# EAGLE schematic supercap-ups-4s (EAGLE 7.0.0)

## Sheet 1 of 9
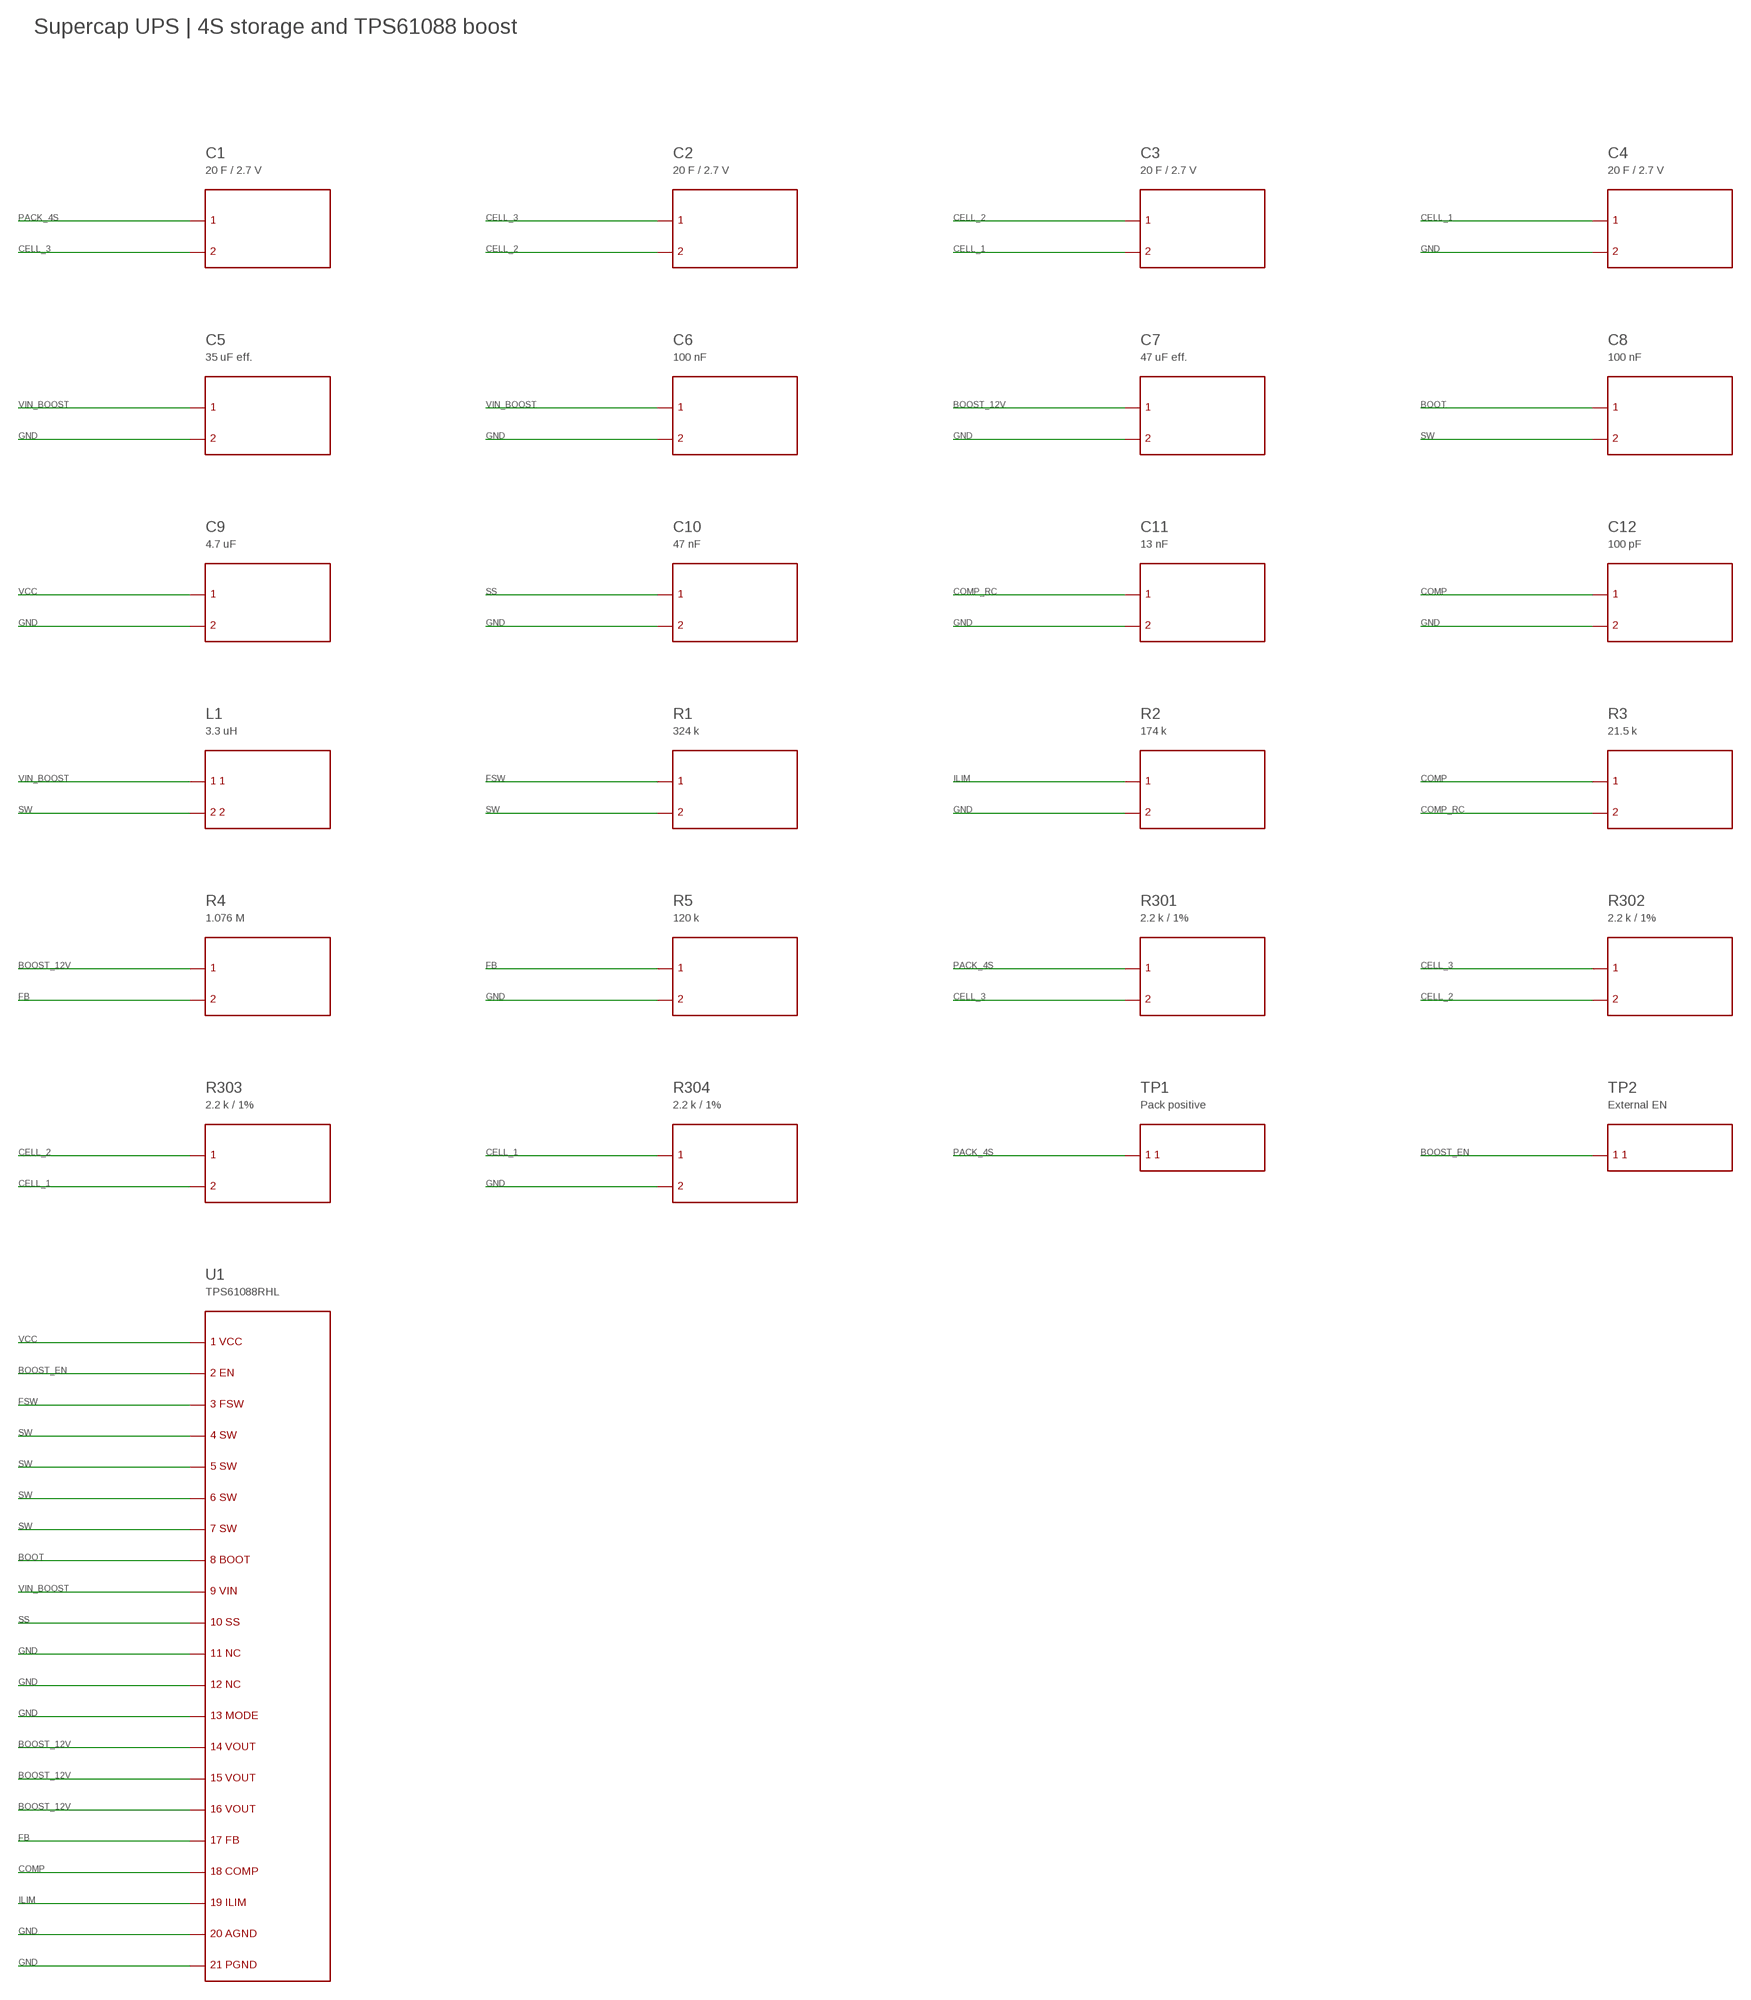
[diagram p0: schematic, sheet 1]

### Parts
C1  20 F / 2.7 V  SYM12  (no package)
C2  20 F / 2.7 V  SYM12  (no package)
C3  20 F / 2.7 V  SYM12  (no package)
C4  20 F / 2.7 V  SYM12  (no package)
C5  35 uF eff.  SYM11  (no package)
C6  100 nF  SYM11  (no package)
C7  47 uF eff.  SYM11  (no package)
C8  100 nF  SYM11  (no package)
C9  4.7 uF  SYM11  (no package)
C10  47 nF  SYM11  (no package)
C11  13 nF  SYM11  (no package)
C12  100 pF  SYM11  (no package)
L1  3.3 uH  SYM14  (no package)
R1  324 k  SYM15  (no package)
R2  174 k  SYM15  (no package)
R3  21.5 k  SYM15  (no package)
R4  1.076 M  SYM15  (no package)
R5  120 k  SYM15  (no package)
R301  2.2 k / 1%  SYM15  (no package)
R302  2.2 k / 1%  SYM15  (no package)
R303  2.2 k / 1%  SYM15  (no package)
R304  2.2 k / 1%  SYM15  (no package)
TP1  Pack positive  SYM8  (no package)
TP2  External EN  SYM8  (no package)
U1  TPS61088RHL  SYM25  (no package)

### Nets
BOOST_12V: C7.P1 R4.P1 U1.P14 U1.P15 U1.P16
BOOST_EN: TP2.P1 U1.P2 ; also sheet 9
BOOT: C8.P1 U1.P8
CELL_1: C3.P2 C4.P1 R303.P2 R304.P1 ; also sheet 4,8
CELL_2: C2.P2 C3.P1 R302.P2 R303.P1 ; also sheet 4,8
CELL_3: C1.P2 C2.P1 R301.P2 R302.P1 ; also sheet 4,8
COMP: C12.P1 R3.P1 U1.P18
COMP_RC: C11.P1 R3.P2
FB: R4.P2 R5.P1 U1.P17
FSW: R1.P1 U1.P3
GND: C4.P2 C5.P2 C6.P2 C7.P2 C9.P2 C10.P2 C11.P2 C12.P2 R2.P2 R5.P2 R304.P2 U1.P11 U1.P12 U1.P13 U1.P20 U1.P21 ; also sheet 2,3,4,5,6,7,8,9
ILIM: R2.P1 U1.P19
PACK_4S: C1.P1 R301.P1 TP1.P1 ; also sheet 2,3,4,5,6,8
SS: C10.P1 U1.P10
SW: C8.P2 L1.P2 R1.P2 U1.P4 U1.P5 U1.P6 U1.P7
VCC: C9.P1 U1.P1
VIN_BOOST: C5.P1 C6.P1 L1.P1 U1.P9 ; also sheet 5

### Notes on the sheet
- Supercap UPS | 4S storage and TPS61088 boost

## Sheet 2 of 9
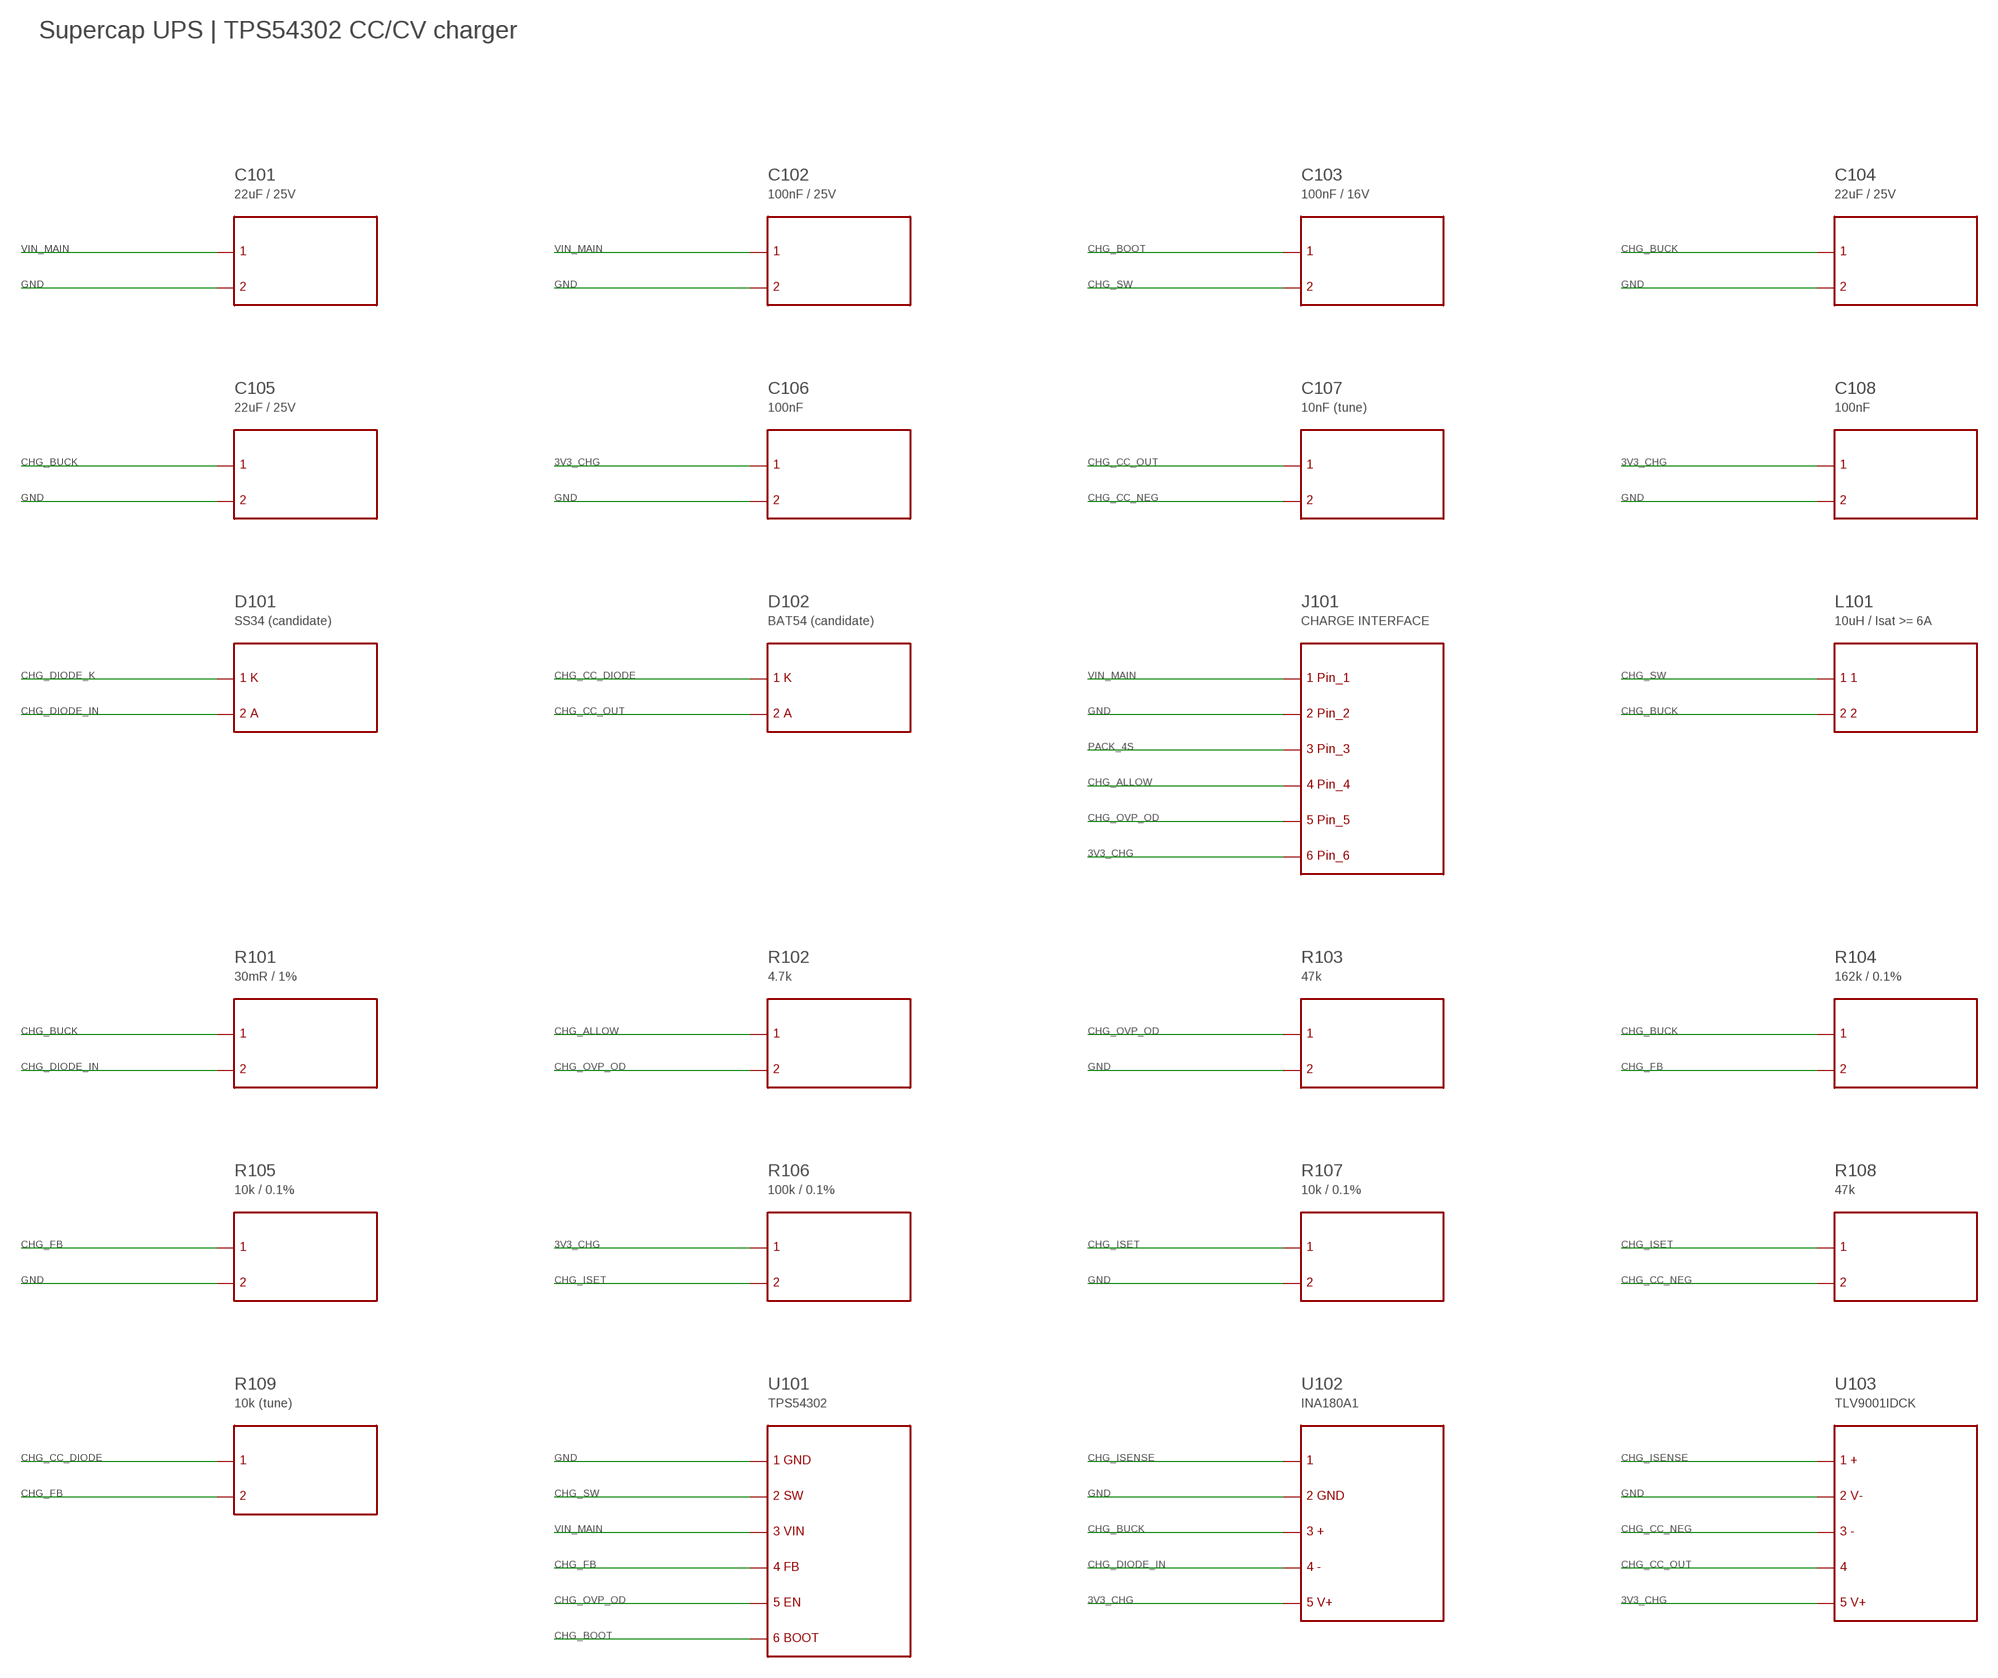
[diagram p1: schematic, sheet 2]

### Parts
C101  22uF / 25V  SYM11  (no package)
C102  100nF / 25V  SYM11  (no package)
C103  100nF / 16V  SYM11  (no package)
C104  22uF / 25V  SYM11  (no package)
C105  22uF / 25V  SYM11  (no package)
C106  100nF  SYM11  (no package)
C107  10nF (tune)  SYM11  (no package)
C108  100nF  SYM11  (no package)
D101  SS34 (candidate)  SYM13  (no package)
D102  BAT54 (candidate)  SYM13  (no package)
J101  CHARGE INTERFACE  SYM9  (no package)
L101  10uH / Isat >= 6A  SYM14  (no package)
R101  30mR / 1%  SYM15  (no package)
R102  4.7k  SYM15  (no package)
R103  47k  SYM15  (no package)
R104  162k / 0.1%  SYM15  (no package)
R105  10k / 0.1%  SYM15  (no package)
R106  100k / 0.1%  SYM15  (no package)
R107  10k / 0.1%  SYM15  (no package)
R108  47k  SYM15  (no package)
R109  10k (tune)  SYM15  (no package)
U101  TPS54302  SYM24  (no package)
U102  INA180A1  SYM0  (no package)
U103  TLV9001IDCK  SYM3  (no package)

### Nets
3V3_CHG: C106.P1 C108.P1 J101.P6 R106.P1 U102.P5 U103.P5 ; also sheet 7
CHG_ALLOW: J101.P4 R102.P1
CHG_BOOT: C103.P1 U101.P6
CHG_BUCK: C104.P1 C105.P1 L101.P2 R101.P1 R104.P1 U102.P3
CHG_CC_DIODE: D102.P1 R109.P1
CHG_CC_NEG: C107.P2 R108.P2 U103.P3
CHG_CC_OUT: C107.P1 D102.P2 U103.P4
CHG_DIODE_IN: D101.P2 R101.P2 U102.P4
CHG_DIODE_K: D101.P1 ; also sheet 6
CHG_FB: R104.P2 R105.P1 R109.P2 U101.P4 ; also sheet 6
CHG_ISENSE: U102.P1 U103.P1
CHG_ISET: R106.P2 R107.P1 R108.P1
CHG_OVP_OD: J101.P5 R102.P2 R103.P1 U101.P5 ; also sheet 4,7
CHG_SW: C103.P2 L101.P1 U101.P2
GND: C101.P2 C102.P2 C104.P2 C105.P2 C106.P2 C108.P2 J101.P2 R103.P2 R105.P2 R107.P2 U101.P1 U102.P2 U103.P2 ; also sheet 1,3,4,5,6,7,8,9
PACK_4S: J101.P3 ; also sheet 1,3,4,5,6,8
VIN_MAIN: C101.P1 C102.P1 J101.P1 U101.P3 ; also sheet 4,7

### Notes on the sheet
- Supercap UPS | TPS54302 CC/CV charger

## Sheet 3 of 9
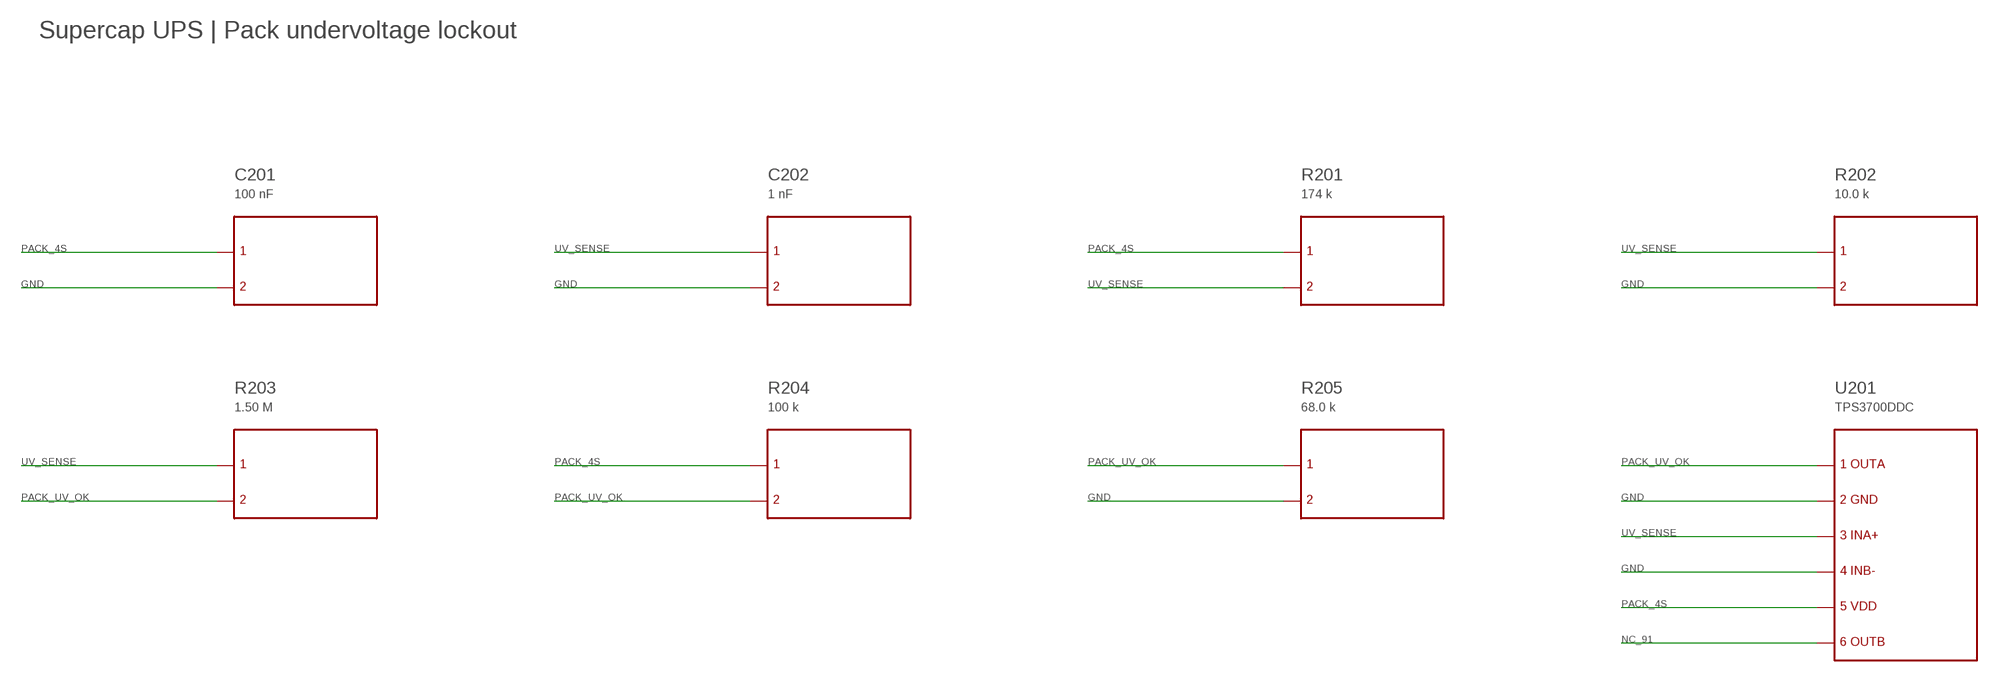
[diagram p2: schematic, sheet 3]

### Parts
C201  100 nF  SYM11  (no package)
C202  1 nF  SYM11  (no package)
R201  174 k  SYM15  (no package)
R202  10.0 k  SYM15  (no package)
R203  1.50 M  SYM15  (no package)
R204  100 k  SYM15  (no package)
R205  68.0 k  SYM15  (no package)
U201  TPS3700DDC  SYM29  (no package)

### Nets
GND: C201.P2 C202.P2 R202.P2 R205.P2 U201.P2 U201.P4 ; also sheet 1,2,4,5,6,7,8,9
NC_91: U201.P6
PACK_4S: C201.P1 R201.P1 R204.P1 U201.P5 ; also sheet 1,2,4,5,6,8
PACK_UV_OK: R203.P2 R204.P2 R205.P1 U201.P1 ; also sheet 5,9
UV_SENSE: C202.P1 R201.P2 R202.P1 R203.P1 U201.P3

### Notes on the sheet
- Supercap UPS | Pack undervoltage lockout

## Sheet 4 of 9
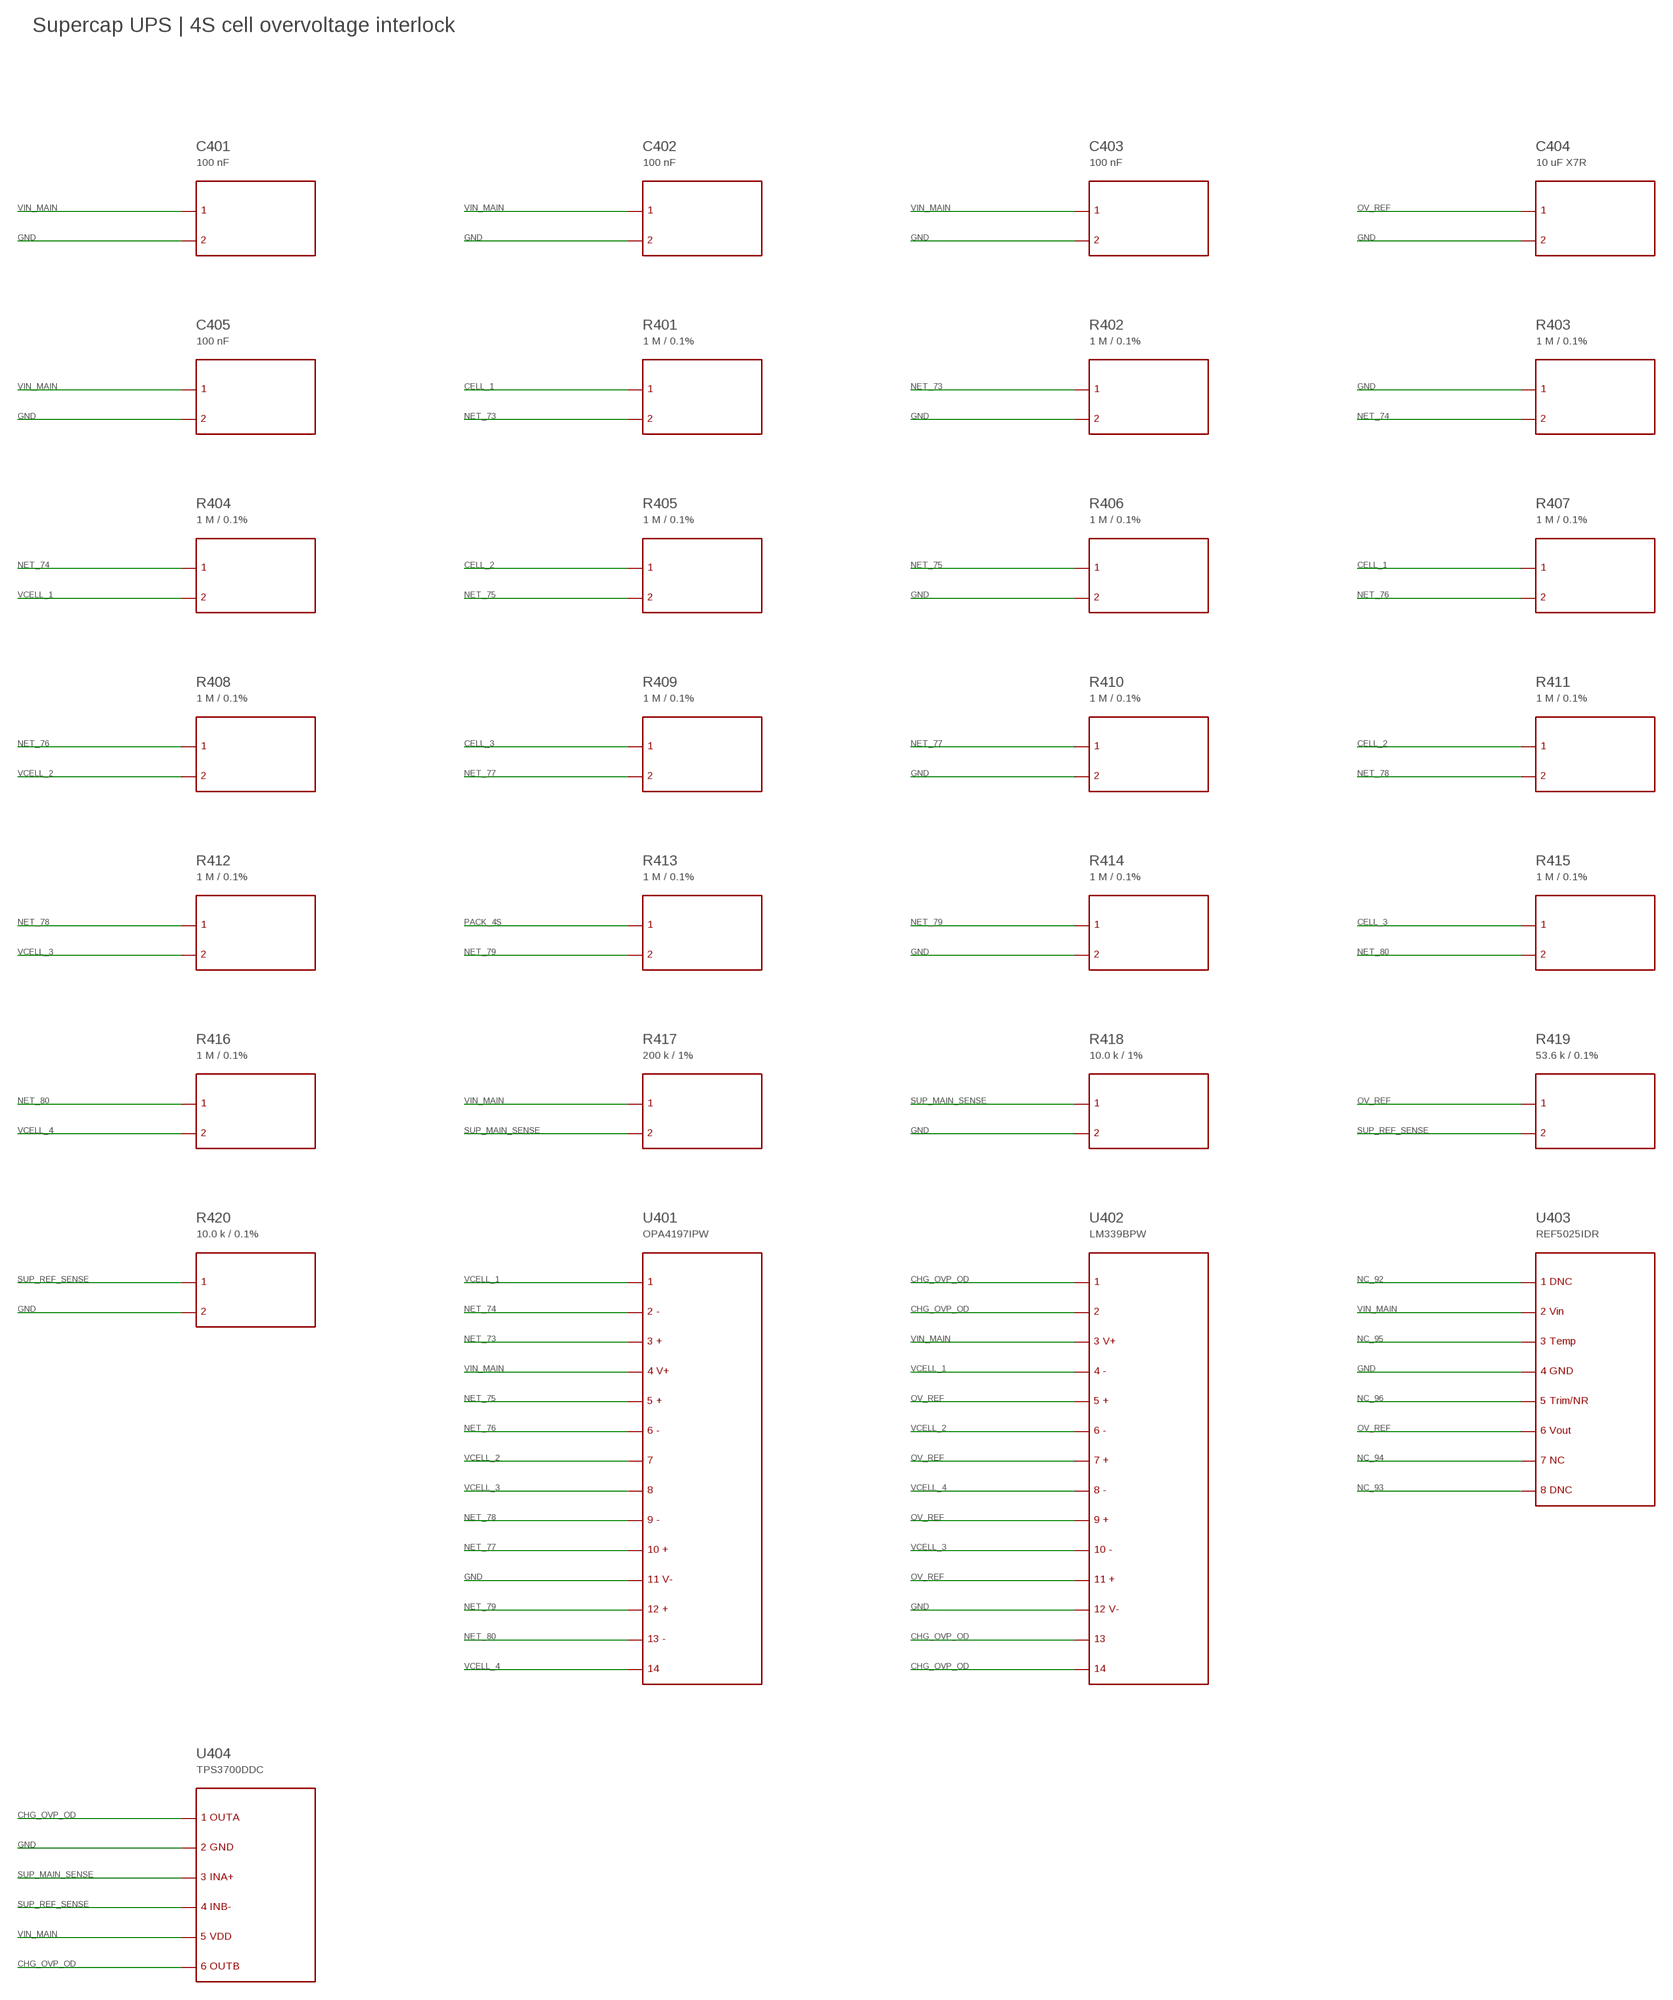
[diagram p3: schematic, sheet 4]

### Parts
C401  100 nF  SYM11  (no package)
C402  100 nF  SYM11  (no package)
C403  100 nF  SYM11  (no package)
C404  10 uF X7R  SYM11  (no package)
C405  100 nF  SYM11  (no package)
R401  1 M / 0.1%  SYM15  (no package)
R402  1 M / 0.1%  SYM15  (no package)
R403  1 M / 0.1%  SYM15  (no package)
R404  1 M / 0.1%  SYM15  (no package)
R405  1 M / 0.1%  SYM15  (no package)
R406  1 M / 0.1%  SYM15  (no package)
R407  1 M / 0.1%  SYM15  (no package)
R408  1 M / 0.1%  SYM15  (no package)
R409  1 M / 0.1%  SYM15  (no package)
R410  1 M / 0.1%  SYM15  (no package)
R411  1 M / 0.1%  SYM15  (no package)
R412  1 M / 0.1%  SYM15  (no package)
R413  1 M / 0.1%  SYM15  (no package)
R414  1 M / 0.1%  SYM15  (no package)
R415  1 M / 0.1%  SYM15  (no package)
R416  1 M / 0.1%  SYM15  (no package)
R417  200 k / 1%  SYM15  (no package)
R418  10.0 k / 1%  SYM15  (no package)
R419  53.6 k / 0.1%  SYM15  (no package)
R420  10.0 k / 0.1%  SYM15  (no package)
U401  OPA4197IPW  SYM2  (no package)
U402  LM339BPW  SYM5  (no package)
U403  REF5025IDR  SYM6  (no package)
U404  TPS3700DDC  SYM7  (no package)

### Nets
CELL_1: R401.P1 R407.P1 ; also sheet 1,8
CELL_2: R405.P1 R411.P1 ; also sheet 1,8
CELL_3: R409.P1 R415.P1 ; also sheet 1,8
CHG_OVP_OD: U402.P1 U402.P2 U402.P13 U402.P14 U404.P1 U404.P6 ; also sheet 2,7
GND: C401.P2 C402.P2 C403.P2 C404.P2 C405.P2 R402.P2 R403.P1 R406.P2 R410.P2 R414.P2 R418.P2 R420.P2 U401.P11 U402.P12 U403.P4 U404.P2 ; also sheet 1,2,3,5,6,7,8,9
NC_92: U403.P1
NC_93: U403.P8
NC_94: U403.P7
NC_95: U403.P3
NC_96: U403.P5
NET_73: R401.P2 R402.P1 U401.P3
NET_74: R403.P2 R404.P1 U401.P2
NET_75: R405.P2 R406.P1 U401.P5
NET_76: R407.P2 R408.P1 U401.P6
NET_77: R409.P2 R410.P1 U401.P10
NET_78: R411.P2 R412.P1 U401.P9
NET_79: R413.P2 R414.P1 U401.P12
NET_80: R415.P2 R416.P1 U401.P13
OV_REF: C404.P1 R419.P1 U402.P5 U402.P7 U402.P9 U402.P11 U403.P6
PACK_4S: R413.P1 ; also sheet 1,2,3,5,6,8
SUP_MAIN_SENSE: R417.P2 R418.P1 U404.P3
SUP_REF_SENSE: R419.P2 R420.P1 U404.P4
VCELL_1: R404.P2 U401.P1 U402.P4
VCELL_2: R408.P2 U401.P7 U402.P6
VCELL_3: R412.P2 U401.P8 U402.P10
VCELL_4: R416.P2 U401.P14 U402.P8
VIN_MAIN: C401.P1 C402.P1 C403.P1 C405.P1 R417.P1 U401.P4 U402.P3 U403.P2 U404.P5 ; also sheet 2,7

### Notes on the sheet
- Supercap UPS | 4S cell overvoltage interlock

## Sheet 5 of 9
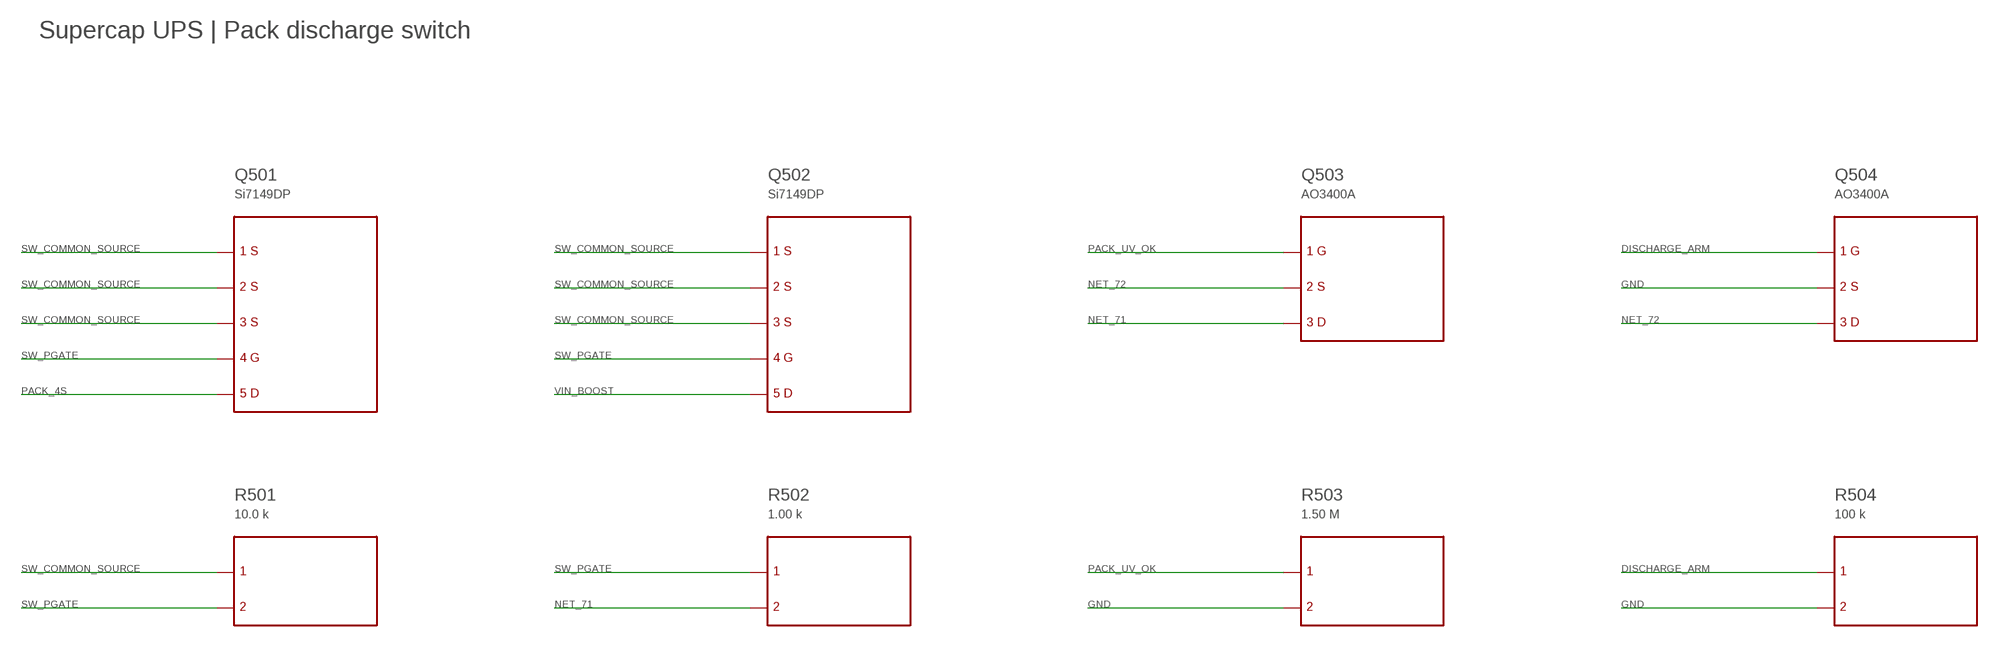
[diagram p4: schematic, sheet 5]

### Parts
Q501  Si7149DP  SYM32  (no package)
Q502  Si7149DP  SYM32  (no package)
Q503  AO3400A  SYM28  (no package)
Q504  AO3400A  SYM28  (no package)
R501  10.0 k  SYM15  (no package)
R502  1.00 k  SYM15  (no package)
R503  1.50 M  SYM15  (no package)
R504  100 k  SYM15  (no package)

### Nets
DISCHARGE_ARM: Q504.P1 R504.P1 ; also sheet 9
GND: Q504.P2 R503.P2 R504.P2 ; also sheet 1,2,3,4,6,7,8,9
NET_71: Q503.P3 R502.P2
NET_72: Q503.P2 Q504.P3
PACK_4S: Q501.P5 ; also sheet 1,2,3,4,6,8
PACK_UV_OK: Q503.P1 R503.P1 ; also sheet 3,9
SW_COMMON_SOURCE: Q501.P1 Q501.P2 Q501.P3 Q502.P1 Q502.P2 Q502.P3 R501.P1
SW_PGATE: Q501.P4 Q502.P4 R501.P2 R502.P1
VIN_BOOST: Q502.P5 ; also sheet 1

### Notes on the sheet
- Supercap UPS | Pack discharge switch

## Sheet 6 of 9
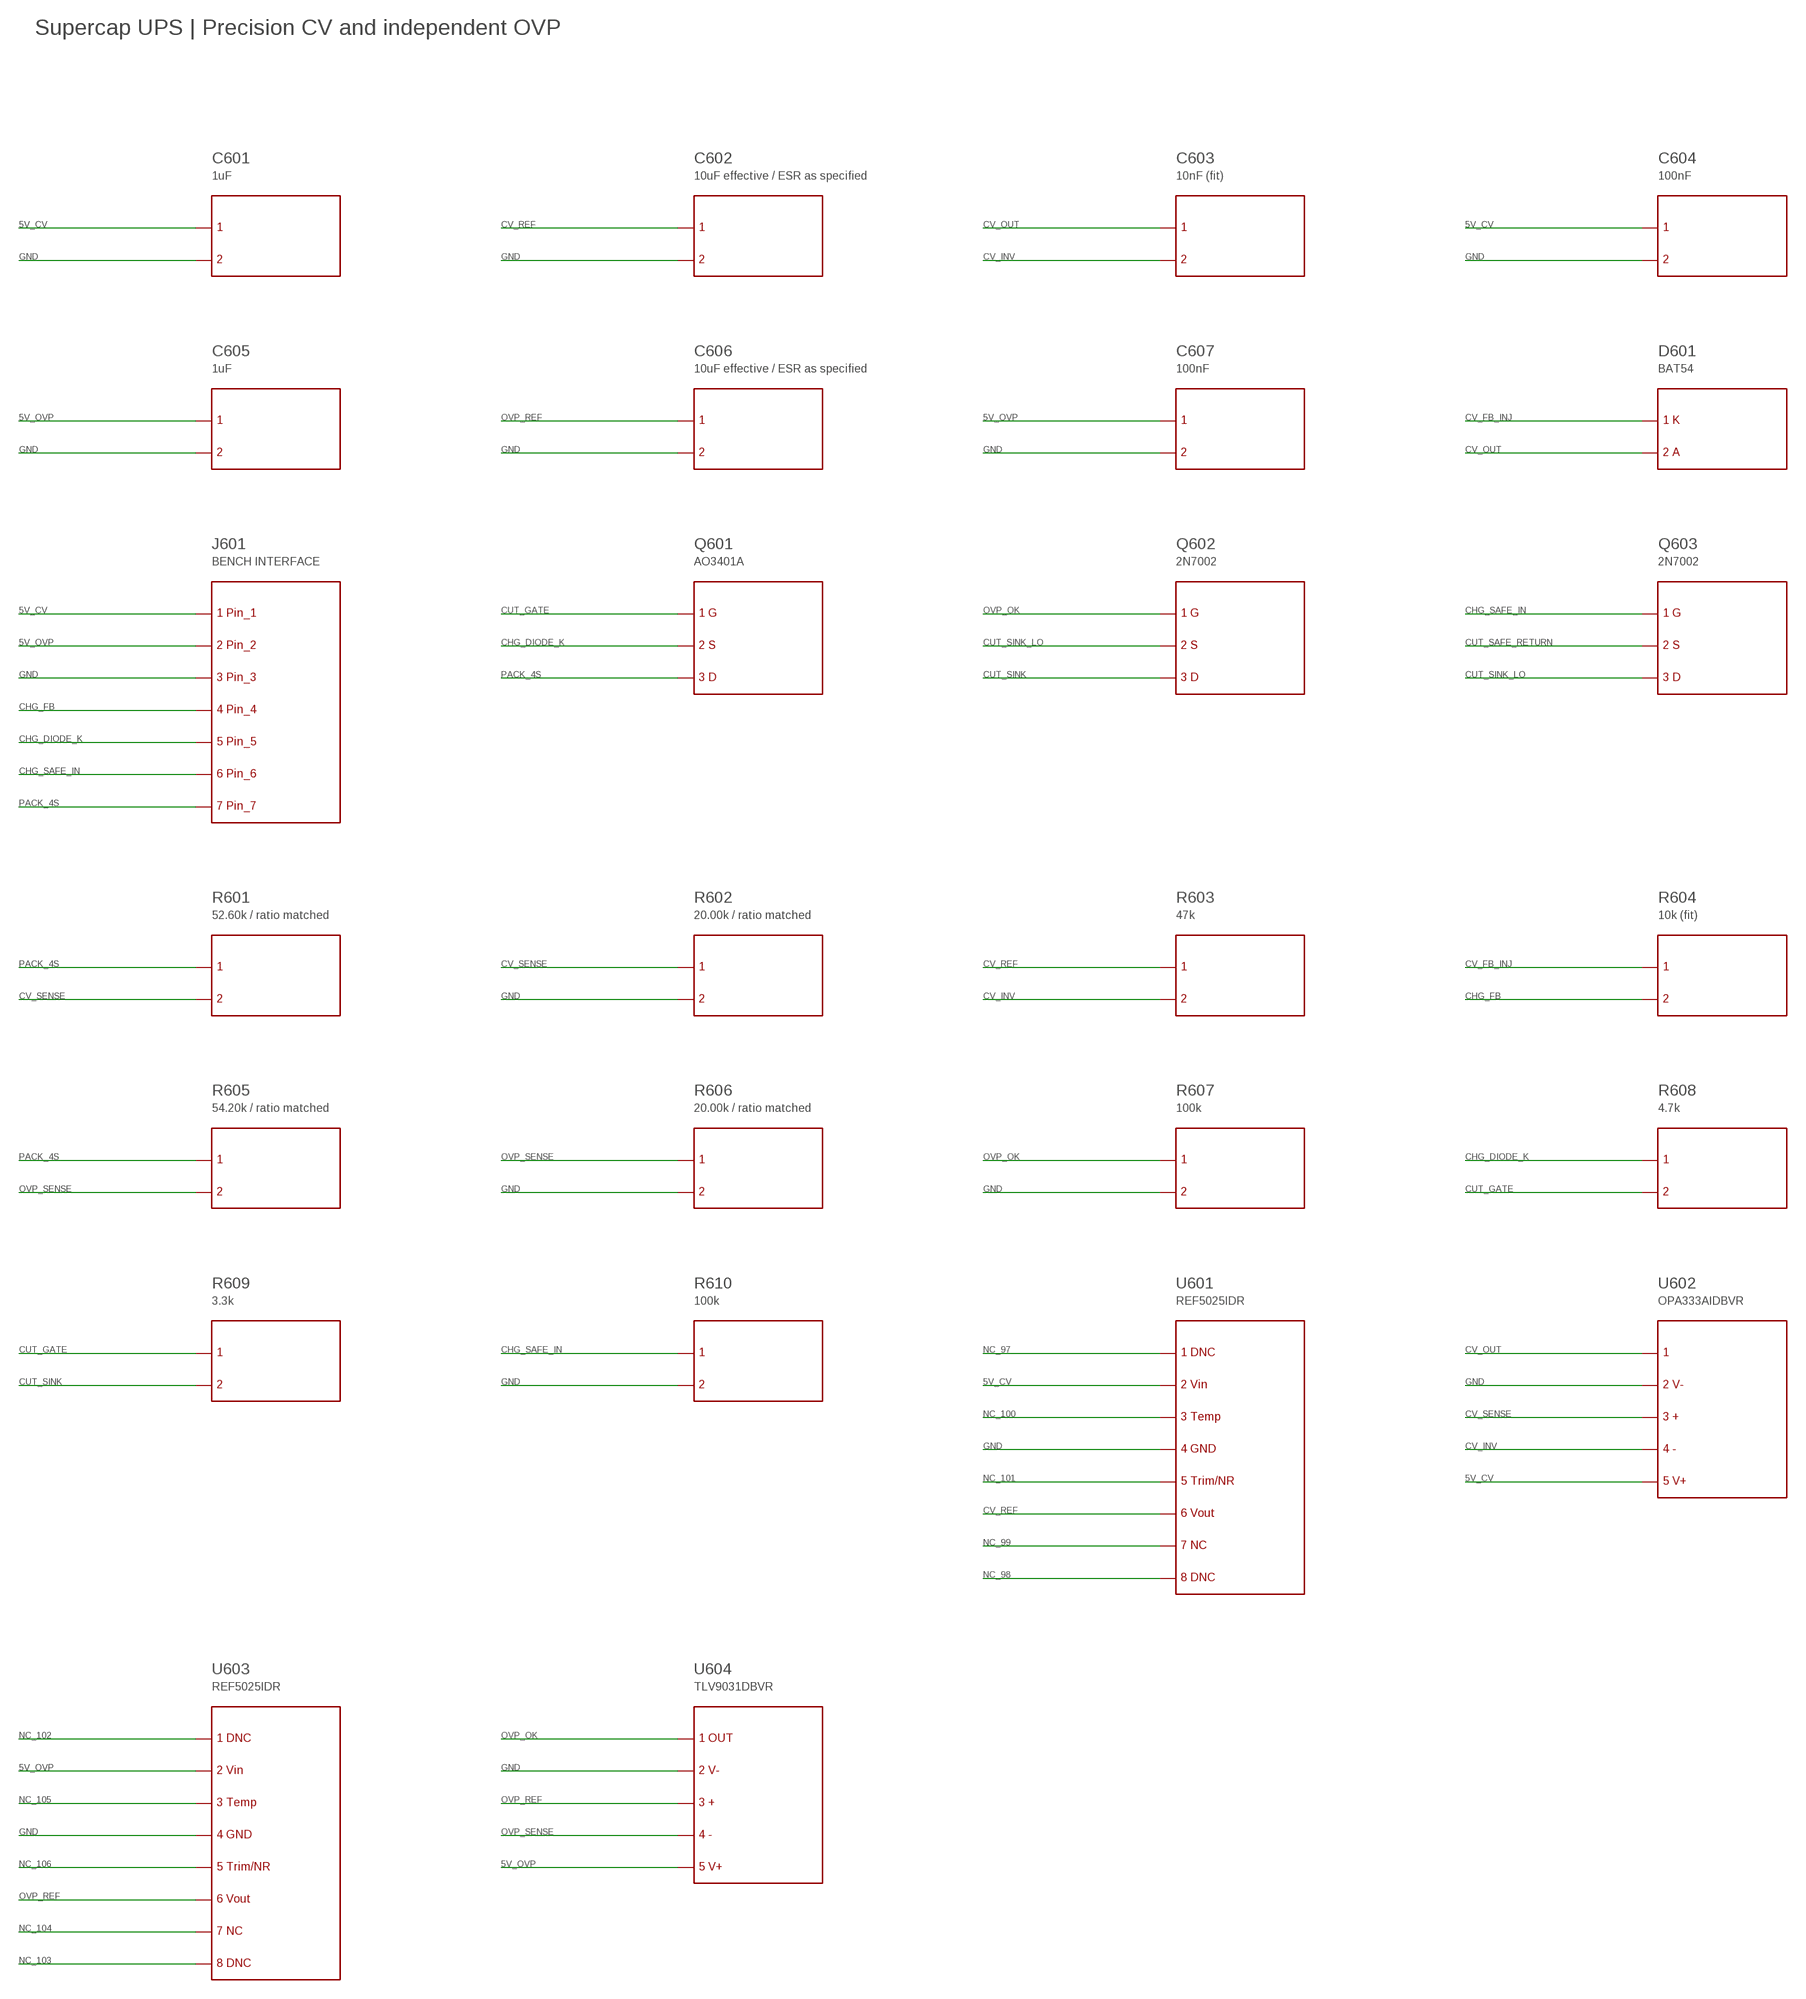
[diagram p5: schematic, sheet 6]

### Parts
C601  1uF  SYM11  (no package)
C602  10uF effective / ESR as specified  SYM11  (no package)
C603  10nF (fit)  SYM11  (no package)
C604  100nF  SYM11  (no package)
C605  1uF  SYM11  (no package)
C606  10uF effective / ESR as specified  SYM11  (no package)
C607  100nF  SYM11  (no package)
D601  BAT54  SYM13  (no package)
J601  BENCH INTERFACE  SYM10  (no package)
Q601  AO3401A  SYM27  (no package)
Q602  2N7002  SYM26  (no package)
Q603  2N7002  SYM26  (no package)
R601  52.60k / ratio matched  SYM15  (no package)
R602  20.00k / ratio matched  SYM15  (no package)
R603  47k  SYM15  (no package)
R604  10k (fit)  SYM15  (no package)
R605  54.20k / ratio matched  SYM15  (no package)
R606  20.00k / ratio matched  SYM15  (no package)
R607  100k  SYM15  (no package)
R608  4.7k  SYM15  (no package)
R609  3.3k  SYM15  (no package)
R610  100k  SYM15  (no package)
U601  REF5025IDR  SYM23  (no package)
U602  OPA333AIDBVR  SYM1  (no package)
U603  REF5025IDR  SYM23  (no package)
U604  TLV9031DBVR  SYM22  (no package)

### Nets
5V_CV: C601.P1 C604.P1 J601.P1 U601.P2 U602.P5 ; also sheet 7
5V_OVP: C605.P1 C607.P1 J601.P2 U603.P2 U604.P5 ; also sheet 7
CHG_DIODE_K: J601.P5 Q601.P2 R608.P1 ; also sheet 2
CHG_FB: J601.P4 R604.P2 ; also sheet 2
CHG_SAFE_IN: J601.P6 Q603.P1 R610.P1
CUT_GATE: Q601.P1 R608.P2 R609.P1
CUT_SAFE_RETURN: Q603.P2 ; also sheet 7
CUT_SINK: Q602.P3 R609.P2
CUT_SINK_LO: Q602.P2 Q603.P3
CV_FB_INJ: D601.P1 R604.P1
CV_INV: C603.P2 R603.P2 U602.P4
CV_OUT: C603.P1 D601.P2 U602.P1
CV_REF: C602.P1 R603.P1 U601.P6
CV_SENSE: R601.P2 R602.P1 U602.P3
GND: C601.P2 C602.P2 C604.P2 C605.P2 C606.P2 C607.P2 J601.P3 R602.P2 R606.P2 R607.P2 R610.P2 U601.P4 U602.P2 U603.P4 U604.P2 ; also sheet 1,2,3,4,5,7,8,9
NC_97: U601.P1
NC_98: U601.P8
NC_99: U601.P7
NC_100: U601.P3
NC_101: U601.P5
NC_102: U603.P1
NC_103: U603.P8
NC_104: U603.P7
NC_105: U603.P3
NC_106: U603.P5
OVP_OK: Q602.P1 R607.P1 U604.P1
OVP_REF: C606.P1 U603.P6 U604.P3
OVP_SENSE: R605.P2 R606.P1 U604.P4
PACK_4S: J601.P7 Q601.P3 R601.P1 R605.P1 ; also sheet 1,2,3,4,5,8

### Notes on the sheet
- Supercap UPS | Precision CV and independent OVP

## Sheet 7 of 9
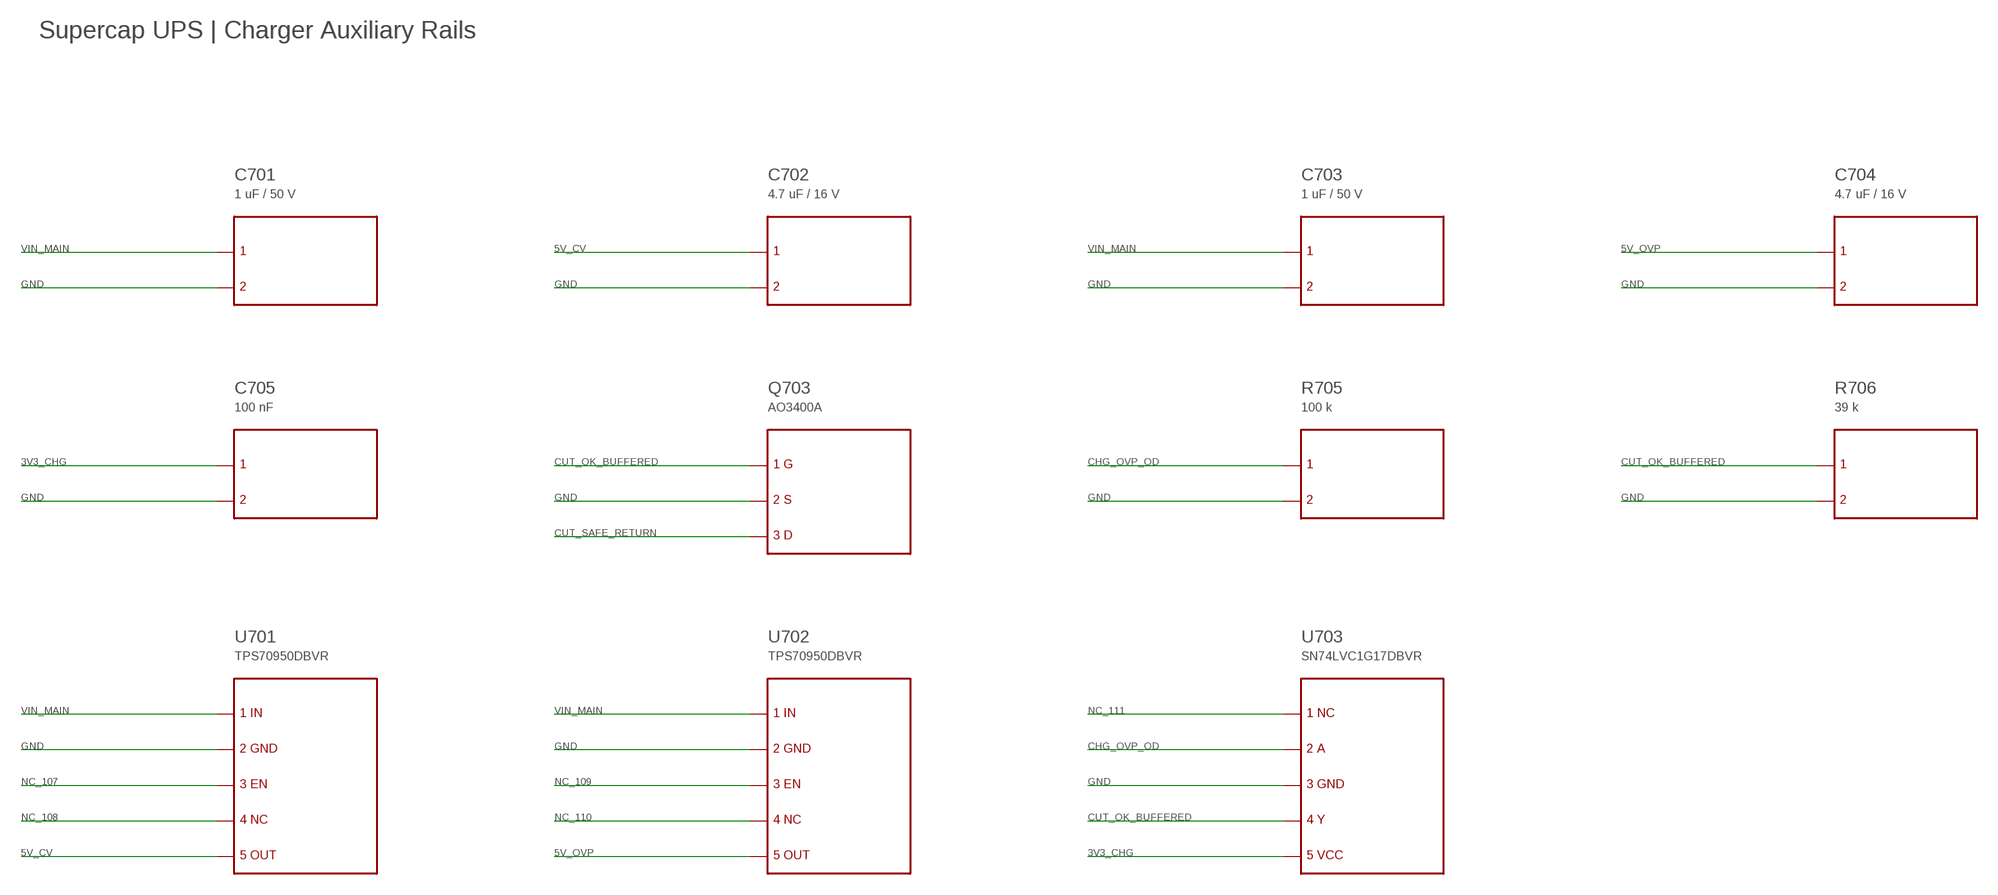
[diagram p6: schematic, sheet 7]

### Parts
C701  1 uF / 50 V  SYM11  (no package)
C702  4.7 uF / 16 V  SYM11  (no package)
C703  1 uF / 50 V  SYM11  (no package)
C704  4.7 uF / 16 V  SYM11  (no package)
C705  100 nF  SYM11  (no package)
Q703  AO3400A  SYM28  (no package)
R705  100 k  SYM15  (no package)
R706  39 k  SYM15  (no package)
U701  TPS70950DBVR  SYM31  (no package)
U702  TPS70950DBVR  SYM31  (no package)
U703  SN74LVC1G17DBVR  SYM30  (no package)

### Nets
3V3_CHG: C705.P1 U703.P5 ; also sheet 2
5V_CV: C702.P1 U701.P5 ; also sheet 6
5V_OVP: C704.P1 U702.P5 ; also sheet 6
CHG_OVP_OD: R705.P1 U703.P2 ; also sheet 2,4
CUT_OK_BUFFERED: Q703.P1 R706.P1 U703.P4
CUT_SAFE_RETURN: Q703.P3 ; also sheet 6
GND: C701.P2 C702.P2 C703.P2 C704.P2 C705.P2 Q703.P2 R705.P2 R706.P2 U701.P2 U702.P2 U703.P3 ; also sheet 1,2,3,4,5,6,8,9
NC_107: U701.P3
NC_108: U701.P4
NC_109: U702.P3
NC_110: U702.P4
NC_111: U703.P1
VIN_MAIN: C701.P1 C703.P1 U701.P1 U702.P1 ; also sheet 2,4

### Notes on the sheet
- Supercap UPS | Charger Auxiliary Rails

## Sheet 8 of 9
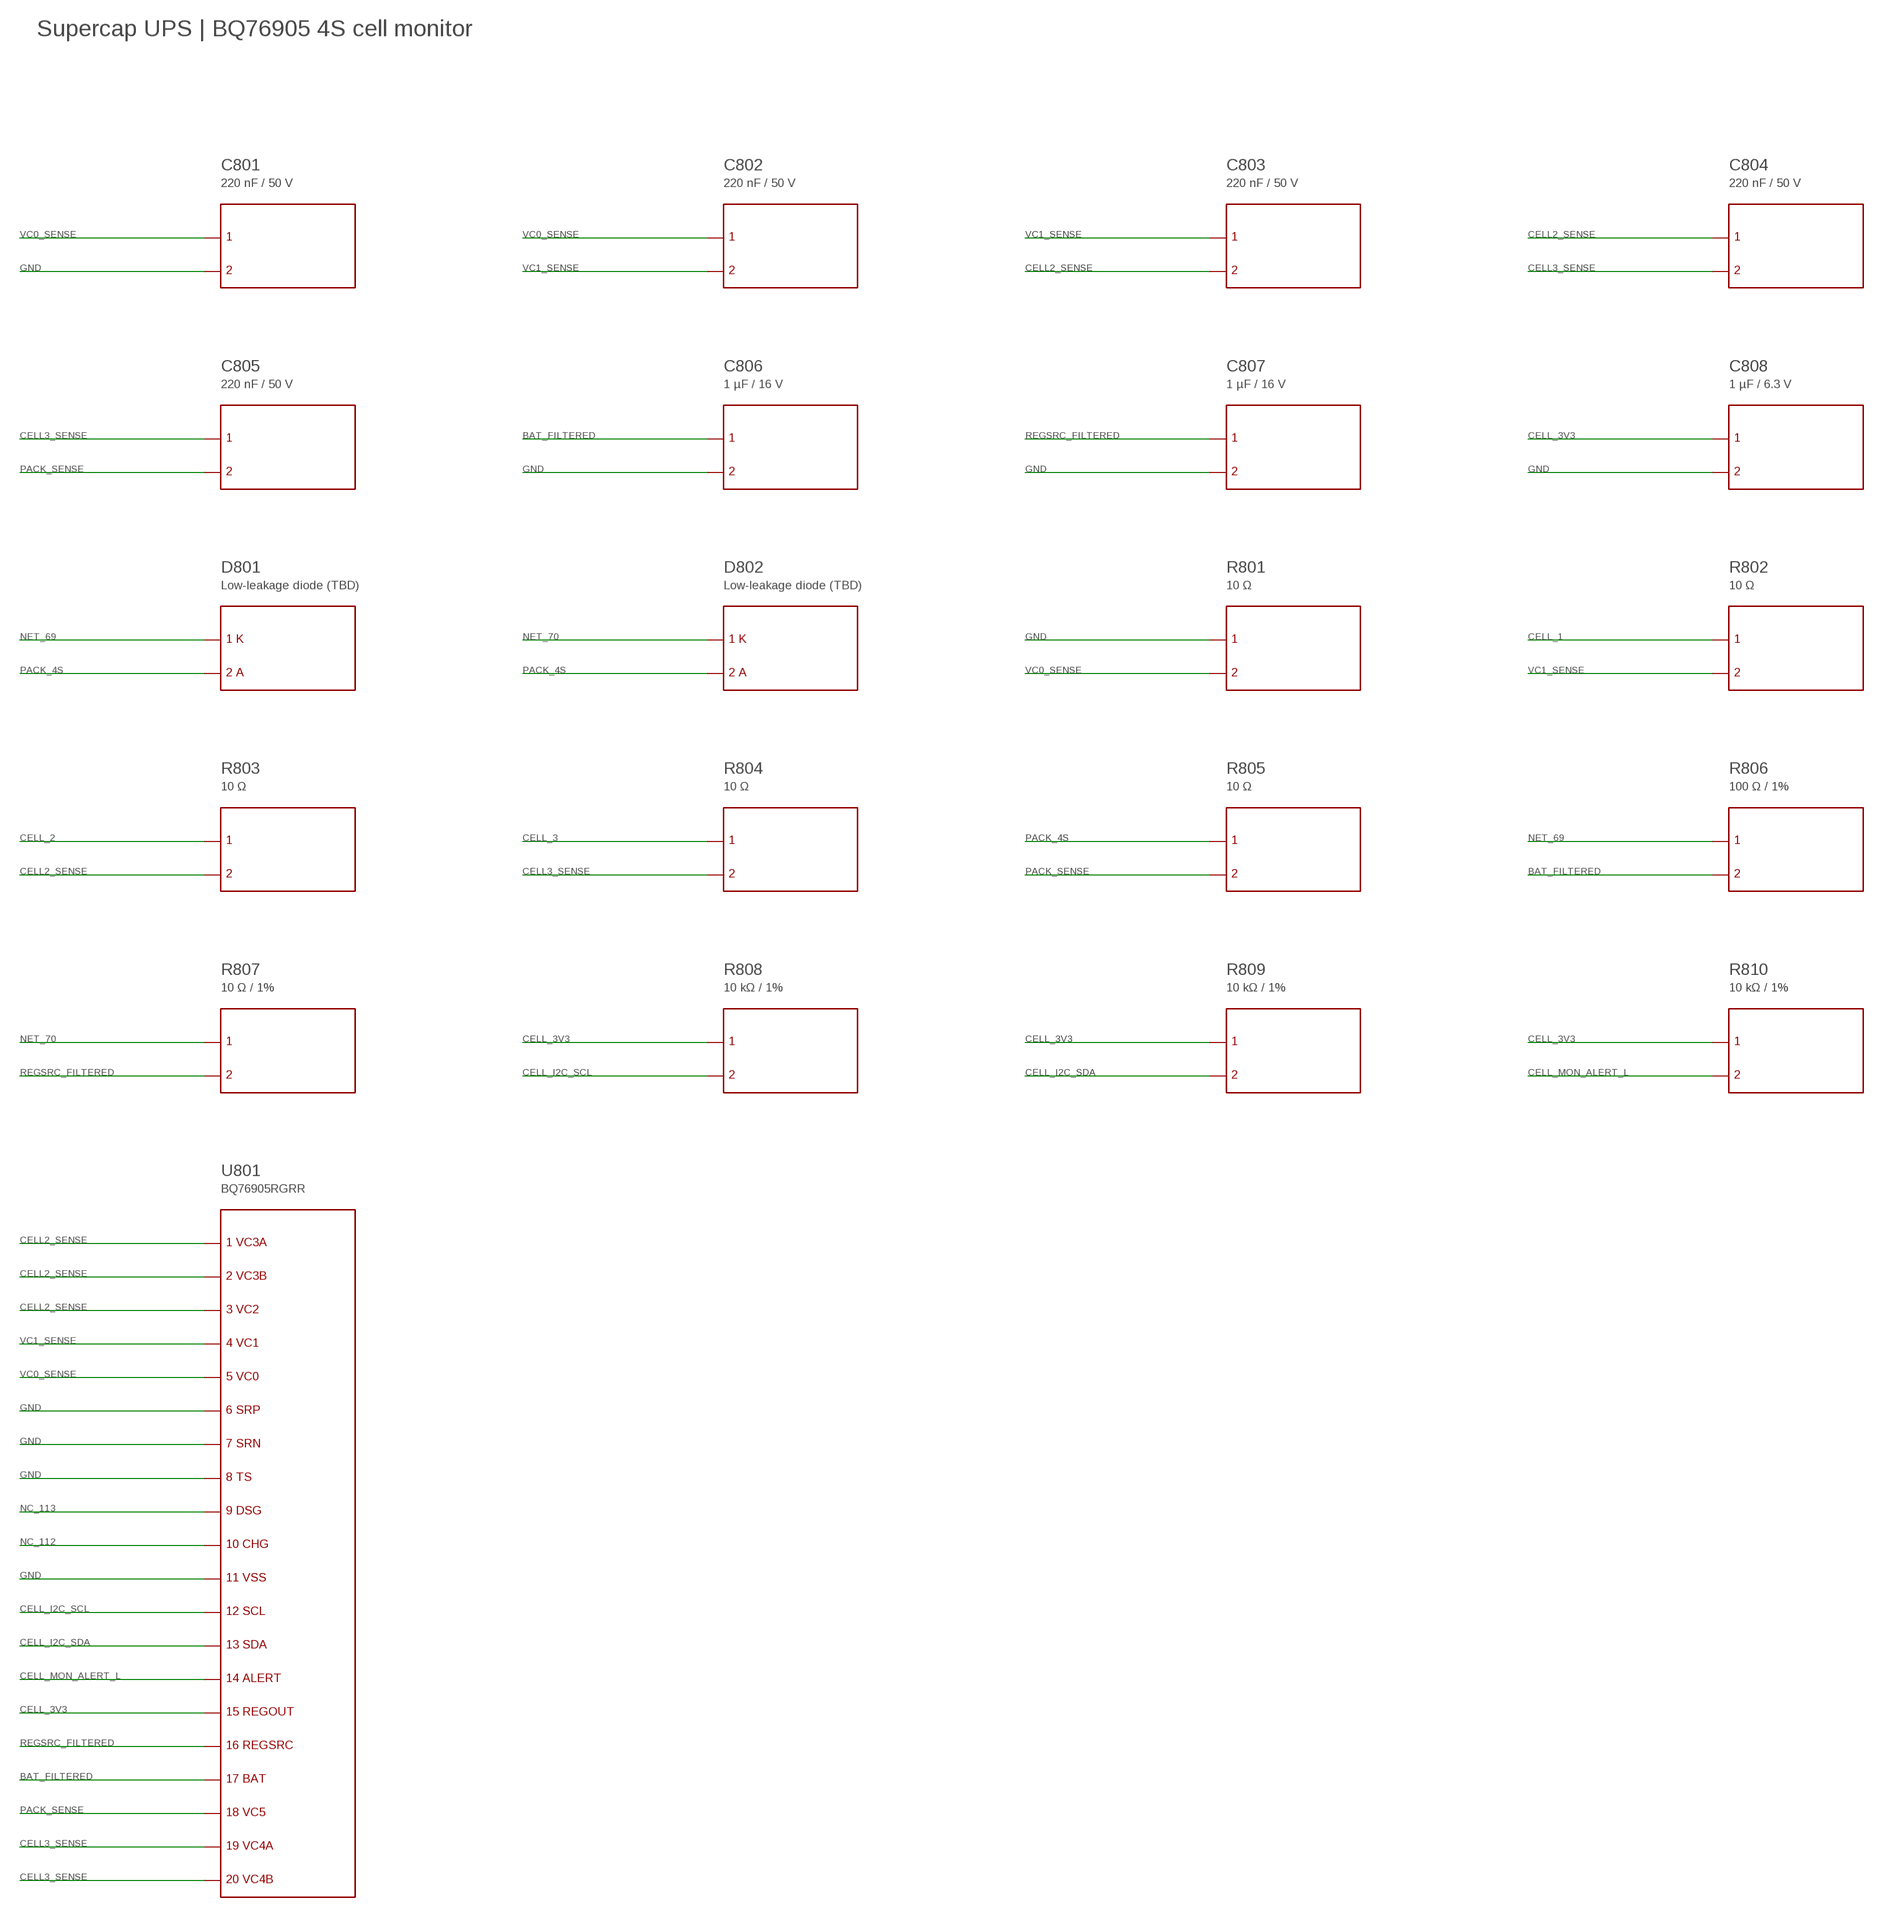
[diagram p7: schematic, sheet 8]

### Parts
C801  220 nF / 50 V  SYM11  (no package)
C802  220 nF / 50 V  SYM11  (no package)
C803  220 nF / 50 V  SYM11  (no package)
C804  220 nF / 50 V  SYM11  (no package)
C805  220 nF / 50 V  SYM11  (no package)
C806  1 µF / 16 V  SYM11  (no package)
C807  1 µF / 16 V  SYM11  (no package)
C808  1 µF / 6.3 V  SYM11  (no package)
D801  Low-leakage diode (TBD)  SYM13  (no package)
D802  Low-leakage diode (TBD)  SYM13  (no package)
R801  10 Ω  SYM15  (no package)
R802  10 Ω  SYM15  (no package)
R803  10 Ω  SYM15  (no package)
R804  10 Ω  SYM15  (no package)
R805  10 Ω  SYM15  (no package)
R806  100 Ω / 1%  SYM15  (no package)
R807  10 Ω / 1%  SYM15  (no package)
R808  10 kΩ / 1%  SYM15  (no package)
R809  10 kΩ / 1%  SYM15  (no package)
R810  10 kΩ / 1%  SYM15  (no package)
U801  BQ76905RGRR  SYM4  (no package)

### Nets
BAT_FILTERED: C806.P1 R806.P2 U801.P17
CELL2_SENSE: C803.P2 C804.P1 R803.P2 U801.P1 U801.P2 U801.P3
CELL3_SENSE: C804.P2 C805.P1 R804.P2 U801.P19 U801.P20
CELL_1: R802.P1 ; also sheet 1,4
CELL_2: R803.P1 ; also sheet 1,4
CELL_3: R804.P1 ; also sheet 1,4
CELL_3V3: C808.P1 R808.P1 R809.P1 R810.P1 U801.P15 ; also sheet 9
CELL_I2C_SCL: R808.P2 U801.P12
CELL_I2C_SDA: R809.P2 U801.P13
CELL_MON_ALERT_L: R810.P2 U801.P14 ; also sheet 9
GND: C801.P2 C806.P2 C807.P2 C808.P2 R801.P1 U801.P6 U801.P7 U801.P8 U801.P11 ; also sheet 1,2,3,4,5,6,7,9
NC_112: U801.P10
NC_113: U801.P9
NET_69: D801.P1 R806.P1
NET_70: D802.P1 R807.P1
PACK_4S: D801.P2 D802.P2 R805.P1 ; also sheet 1,2,3,4,5,6
PACK_SENSE: C805.P2 R805.P2 U801.P18
REGSRC_FILTERED: C807.P1 R807.P2 U801.P16
VC0_SENSE: C801.P1 C802.P1 R801.P2 U801.P5
VC1_SENSE: C802.P2 C803.P1 R802.P2 U801.P4

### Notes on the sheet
- Supercap UPS | BQ76905 4S cell monitor

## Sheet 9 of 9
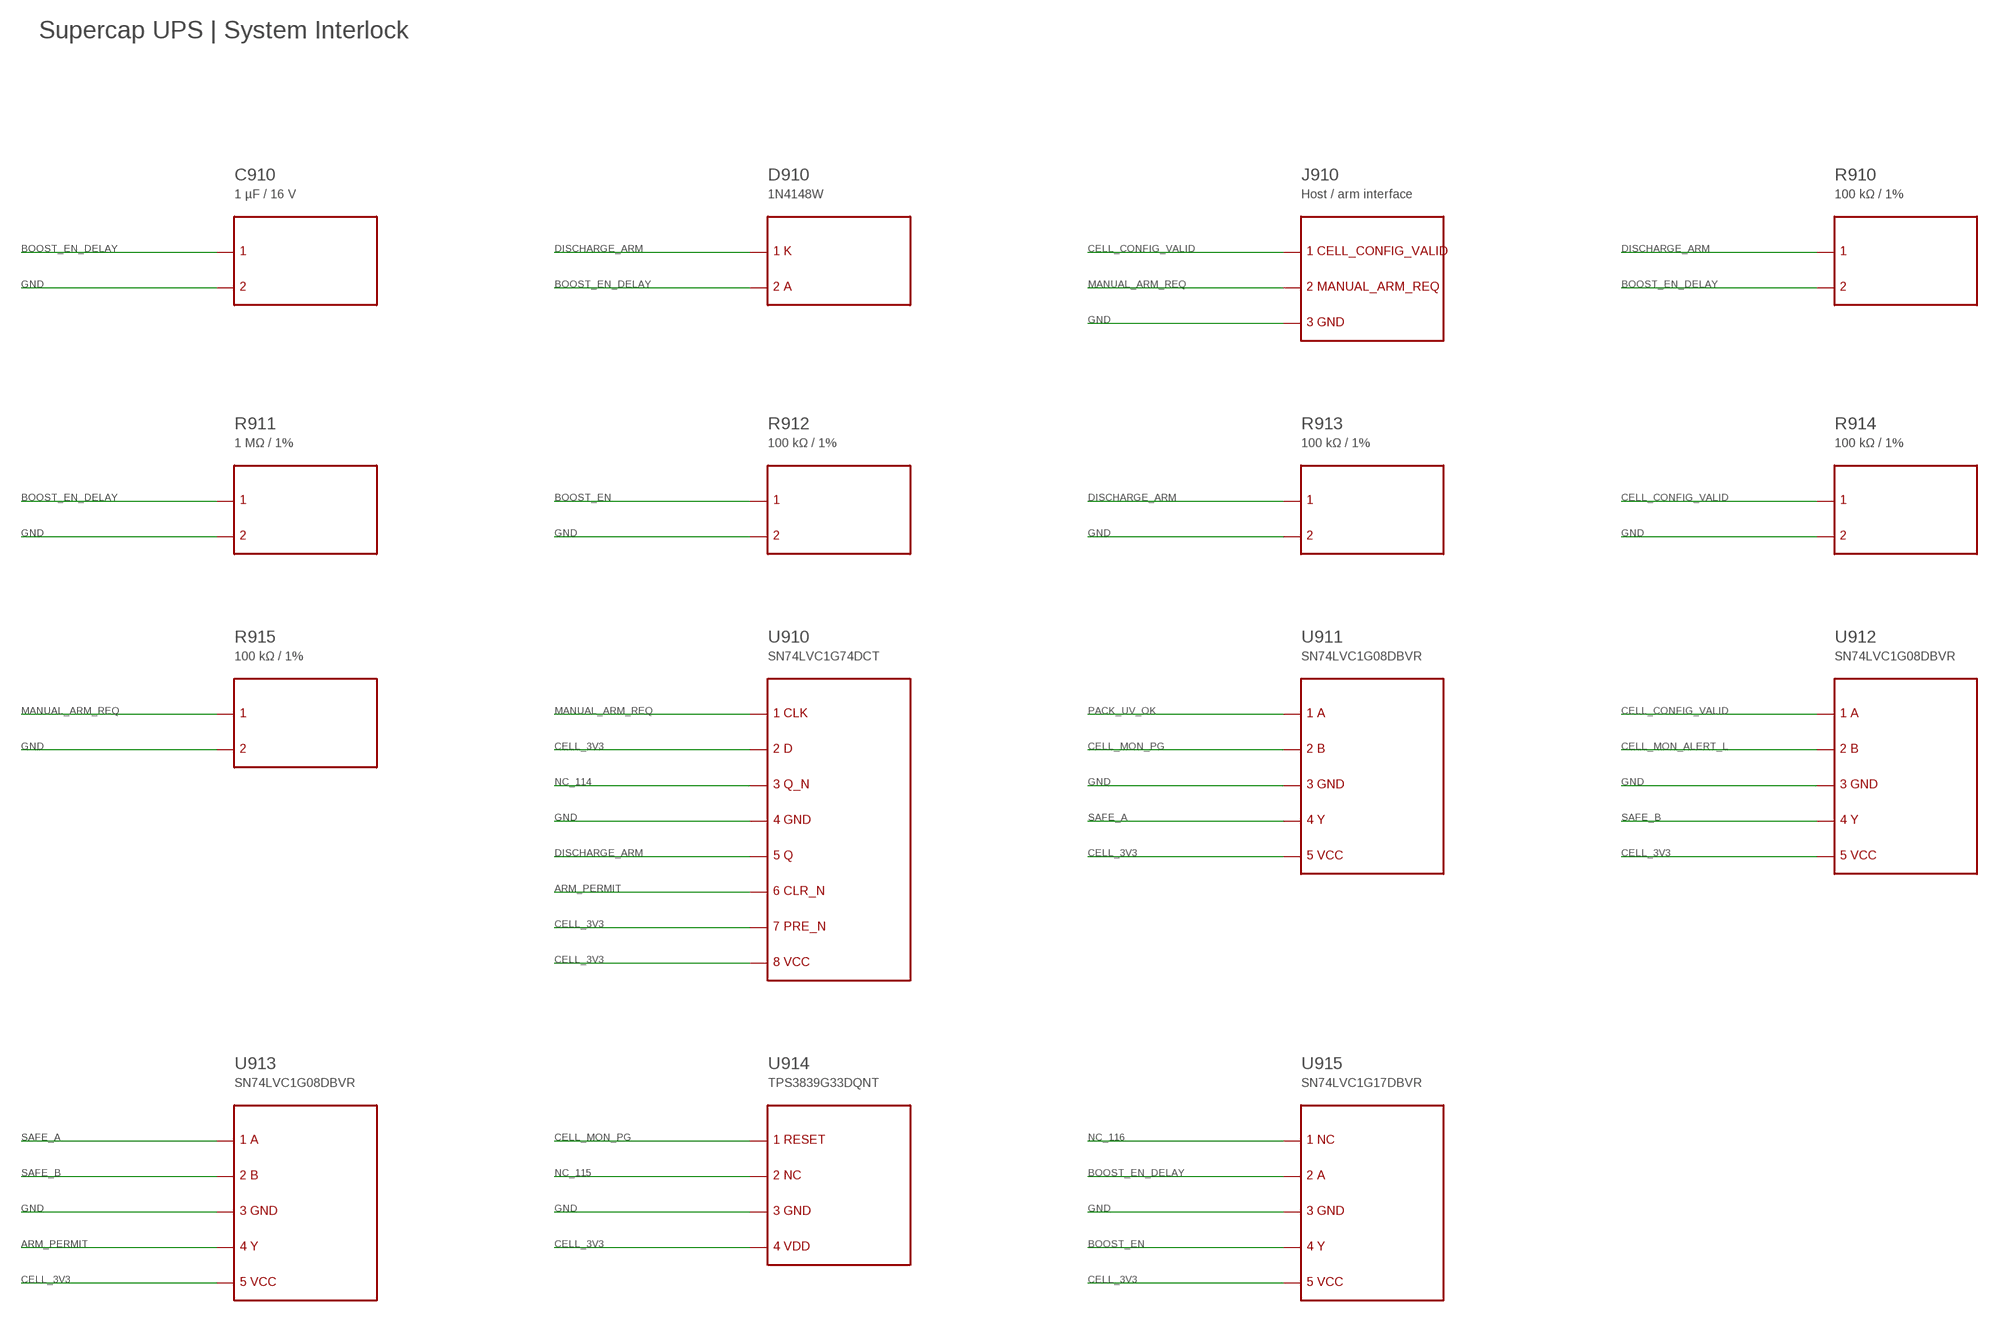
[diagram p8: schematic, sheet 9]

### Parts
C910  1 µF / 16 V  SYM11  (no package)
D910  1N4148W  SYM16  (no package)
J910  Host / arm interface  SYM17  (no package)
R910  100 kΩ / 1%  SYM15  (no package)
R911  1 MΩ / 1%  SYM15  (no package)
R912  100 kΩ / 1%  SYM15  (no package)
R913  100 kΩ / 1%  SYM15  (no package)
R914  100 kΩ / 1%  SYM15  (no package)
R915  100 kΩ / 1%  SYM15  (no package)
U910  SN74LVC1G74DCT  SYM20  (no package)
U911  SN74LVC1G08DBVR  SYM18  (no package)
U912  SN74LVC1G08DBVR  SYM18  (no package)
U913  SN74LVC1G08DBVR  SYM18  (no package)
U914  TPS3839G33DQNT  SYM21  (no package)
U915  SN74LVC1G17DBVR  SYM19  (no package)

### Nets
ARM_PERMIT: U910.P6 U913.P4
BOOST_EN: R912.P1 U915.P4 ; also sheet 1
BOOST_EN_DELAY: C910.P1 D910.P2 R910.P2 R911.P1 U915.P2
CELL_3V3: U910.P2 U910.P7 U910.P8 U911.P5 U912.P5 U913.P5 U914.P4 U915.P5 ; also sheet 8
CELL_CONFIG_VALID: J910.P1 R914.P1 U912.P1
CELL_MON_ALERT_L: U912.P2 ; also sheet 8
CELL_MON_PG: U911.P2 U914.P1
DISCHARGE_ARM: D910.P1 R910.P1 R913.P1 U910.P5 ; also sheet 5
GND: C910.P2 J910.P3 R911.P2 R912.P2 R913.P2 R914.P2 R915.P2 U910.P4 U911.P3 U912.P3 U913.P3 U914.P3 U915.P3 ; also sheet 1,2,3,4,5,6,7,8
MANUAL_ARM_REQ: J910.P2 R915.P1 U910.P1
NC_114: U910.P3
NC_115: U914.P2
NC_116: U915.P1
PACK_UV_OK: U911.P1 ; also sheet 3,5
SAFE_A: U911.P4 U913.P1
SAFE_B: U912.P4 U913.P2

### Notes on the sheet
- Supercap UPS | System Interlock

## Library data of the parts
C1-C4 = UPS:SYM12; SOURCE_FOOTPRINT: Capacitor_THT:CP_Radial_D12.5mm_P5.00mm; SOURCE_MPN: HVH1230-2R7206-R
C5-C12 C101-C108 C201 C202 C601-C607 = UPS:SYM11
C401-C405 C701-C704 C806-C808 C910 = UPS:SYM11; SOURCE_FOOTPRINT: Capacitor_SMD:C_0805_2012Metric
C705 C801-C805 = UPS:SYM11; SOURCE_FOOTPRINT: Capacitor_SMD:C_0603_1608Metric
D101 D102 D601 D801 D802 = UPS:SYM13
D910 = UPS:SYM16; SOURCE_DATASHEET: https://www.vishay.com/docs/81857/1n4148w.pdf; SOURCE_FOOTPRINT: Diode_SMD:D_SOD-323
J101 = UPS:SYM9
J601 = UPS:SYM10
J910 = UPS:SYM17; SOURCE_FOOTPRINT: Connector_PinHeader_2.54mm:PinHeader_1x03_P2.54mm_Vertical
L1 L101 = UPS:SYM14
Q501 Q502 = UPS:SYM32; SOURCE_FOOTPRINT: Package_SO:PowerPAK_SO-8_Single
Q503 Q504 Q703 = UPS:SYM28; SOURCE_FOOTPRINT: Package_TO_SOT_SMD:SOT-23
Q601 = UPS:SYM27; SOURCE_FOOTPRINT: Package_TO_SOT_SMD:SOT-23
Q602 Q603 = UPS:SYM26; SOURCE_FOOTPRINT: Package_TO_SOT_SMD:SOT-23
R1-R5 R101-R109 R201-R205 R501-R504 R601-R610 = UPS:SYM15
R301-R304 R401-R420 = UPS:SYM15; SOURCE_FOOTPRINT: Resistor_SMD:R_0805_2012Metric
R705 R706 R801-R810 R910-R915 = UPS:SYM15; SOURCE_FOOTPRINT: Resistor_SMD:R_0603_1608Metric
TP1 TP2 = UPS:SYM8
U1 = UPS:SYM25
U101 = UPS:SYM24; SOURCE_FOOTPRINT: Package_TO_SOT_SMD:SOT-23-6
U102 = UPS:SYM0; SOURCE_FOOTPRINT: Package_TO_SOT_SMD:SOT-23-5
U103 = UPS:SYM3; SOURCE_FOOTPRINT: Package_TO_SOT_SMD:SOT-353_SC-70-5
U201 = UPS:SYM29; SOURCE_FOOTPRINT: Package_TO_SOT_SMD:SOT-23-6
U401 = UPS:SYM2; SOURCE_FOOTPRINT: Package_SO:TSSOP-14_4.4x5mm_P0.65mm
U402 = UPS:SYM5; SOURCE_FOOTPRINT: Package_SO:TSSOP-14_4.4x5mm_P0.65mm
U403 = UPS:SYM6; SOURCE_FOOTPRINT: Package_SO:SOIC-8_3.9x4.9mm_P1.27mm
U404 = UPS:SYM7; SOURCE_FOOTPRINT: Package_TO_SOT_SMD:SOT-23-6
U601 U603 = UPS:SYM23; SOURCE_FOOTPRINT: Package_SO:SOIC-8_3.9x4.9mm_P1.27mm
U602 = UPS:SYM1; SOURCE_FOOTPRINT: Package_TO_SOT_SMD:SOT-23-5
U604 = UPS:SYM22; SOURCE_FOOTPRINT: Package_TO_SOT_SMD:SOT-23-5
U701 U702 = UPS:SYM31; SOURCE_FOOTPRINT: Package_TO_SOT_SMD:SOT-23-5
U703 = UPS:SYM30; SOURCE_FOOTPRINT: Package_TO_SOT_SMD:SOT-23-5
U801 = UPS:SYM4; SOURCE_DATASHEET: https://www.ti.com/lit/ds/symlink/bq76905.pdf
U910 = UPS:SYM20; SOURCE_DATASHEET: https://www.ti.com/lit/ds/symlink/sn74lvc1g74.pdf; SOURCE_FOOTPRINT: Package_SO:SSOP-8_3x3mm_P0.65mm
U911-U913 = UPS:SYM18; SOURCE_DATASHEET: https://www.ti.com/lit/ds/symlink/sn74lvc1g08.pdf; SOURCE_FOOTPRINT: Package_TO_SOT_SMD:SOT-23-5
U914 = UPS:SYM21; SOURCE_DATASHEET: https://www.ti.com/lit/ds/symlink/tps3839.pdf
U915 = UPS:SYM19; SOURCE_DATASHEET: https://www.ti.com/lit/ds/symlink/sn74lvc1g17.pdf; SOURCE_FOOTPRINT: Package_TO_SOT_SMD:SOT-23-5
